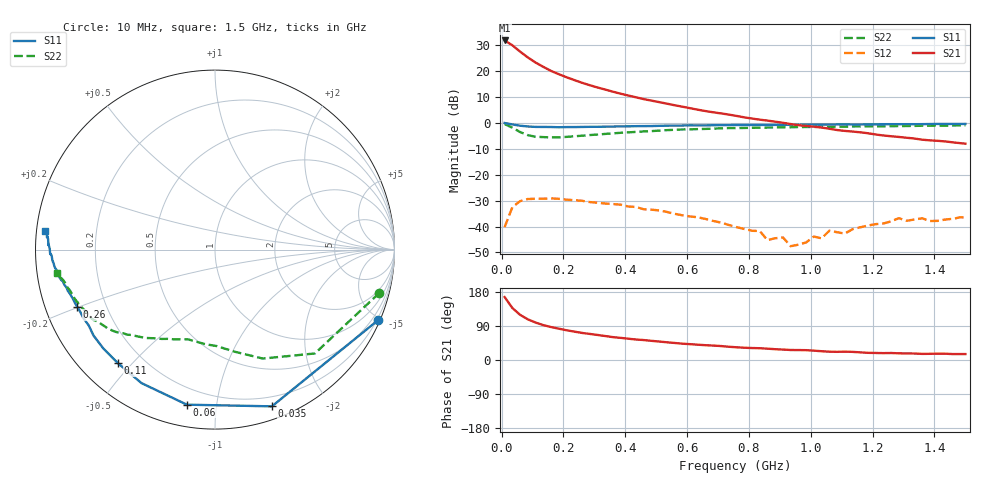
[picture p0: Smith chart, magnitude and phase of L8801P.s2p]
!  POLYFET RF DEVICES
!  L8801P S-PARAMETERS
!  Vds=28.0,Idq=200ma,Vgs=3.01V
# MHZ S MA R 50
! Freq=MHz Mag[s11] Ang[s11] Mag[s21] Ang[s21] Mag[s12] Ang[s12] Mag[s22] Ang[s22]
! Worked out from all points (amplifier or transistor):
!   61 points, 10 MHz to 1.5 GHz, reference 50 ohm
!   highest |S21| = 31.7 dB at 10 MHz (marker M1)
!   |S21| within 3 dB of that: start of sweep to 46.73 MHz
!   unconditionally stable (mu >= 1): 626.2 MHz to end of sweep
!   at 260 MHz: K = 0.23, MSG = 22.8 dB, |S12| = -30.1 dB
!   at 760 MHz: K = 1.84, MAG = 16.1 dB, |S12| = -40.2 dB
!   at 1.5 GHz: K = 2.05, MAG = 8.4 dB, |S12| = -36.6 dB
!   S11 on the Smith chart (normalised r, x): 10 MHz: 0.11, -4.84; 35 MHz: 0.11, -1.42; 60 MHz: 0.11, -0.83; 110 MHz: 0.11, -0.46; 260 MHz: 0.10, -0.20; 1.5 GHz: 0.03, +0.05
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10  0.9907 -23.3  38.65 166.2  0.00972 84.1  0.9462 -14.9
35  0.929 -70.1  31.22 137.3  0.02355 47.8  0.8029 -46.1
60  0.8781 -100.3  23.57 119.2  0.0309 31.0  0.6629 -66.3
85  0.8491 -118.8  18.19 107.3  0.03391 19.4  0.5778 -79.4
110  0.8326 -130.5  14.5 98.9  0.03426 11.2  0.5379 -88.9
135  0.8309 -138.5  11.99 92.1  0.03441 6.7  0.5295 -96.0
160  0.8291 -144.7  10.01 87.0  0.03487 0.6  0.5224 -103.3
210  0.8266 -152.3  7.56 78.5  0.0329 -5.8  0.535 -110.8
260  0.8308 -157.4  5.916 71.5  0.03137 -10.7  0.5631 -118.0
310  0.8365 -160.5  4.798 66.1  0.02878 -14.7  0.5929 -123.5
360  0.846 -163.3  3.975 60.4  0.02708 -18.3  0.6257 -128.1
435  0.8608 -166.7  3.099 54.0  0.02379 -20.3  0.6671 -134.5
510  0.8732 -168.8  2.5 48.7  0.02042 -25.4  0.7067 -138.9
635  0.89 -172.4  1.786 40.3  0.01507 -22.9  0.7554 -146.4
760  0.9063 -175.8  1.355 33.5  0.00975 -14.8  0.791 -152.4
835  0.9083 -176.4  1.149 31.1  0.00818 -7.3  0.8039 -155.6
860  0.9095 -177.2  1.102 29.9  0.00547 -7.3  0.8094 -156.6
910  0.9158 -178.3  0.9994 27.5  0.00616 8.5  0.8183 -158.3
935  0.9167 -178.5  0.9454 26.4  0.00418 20.5  0.8203 -159.1
1010  0.9197 -179.4  0.842 24.7  0.0064 55.9  0.8304 -161.9
1260  0.9369 175.5  0.5498 18.5  0.0126 81.3  0.8599 -168.2
1500  0.9503 173.7  0.3956 15.6  0.01479 99.9  0.8907 -171.7
